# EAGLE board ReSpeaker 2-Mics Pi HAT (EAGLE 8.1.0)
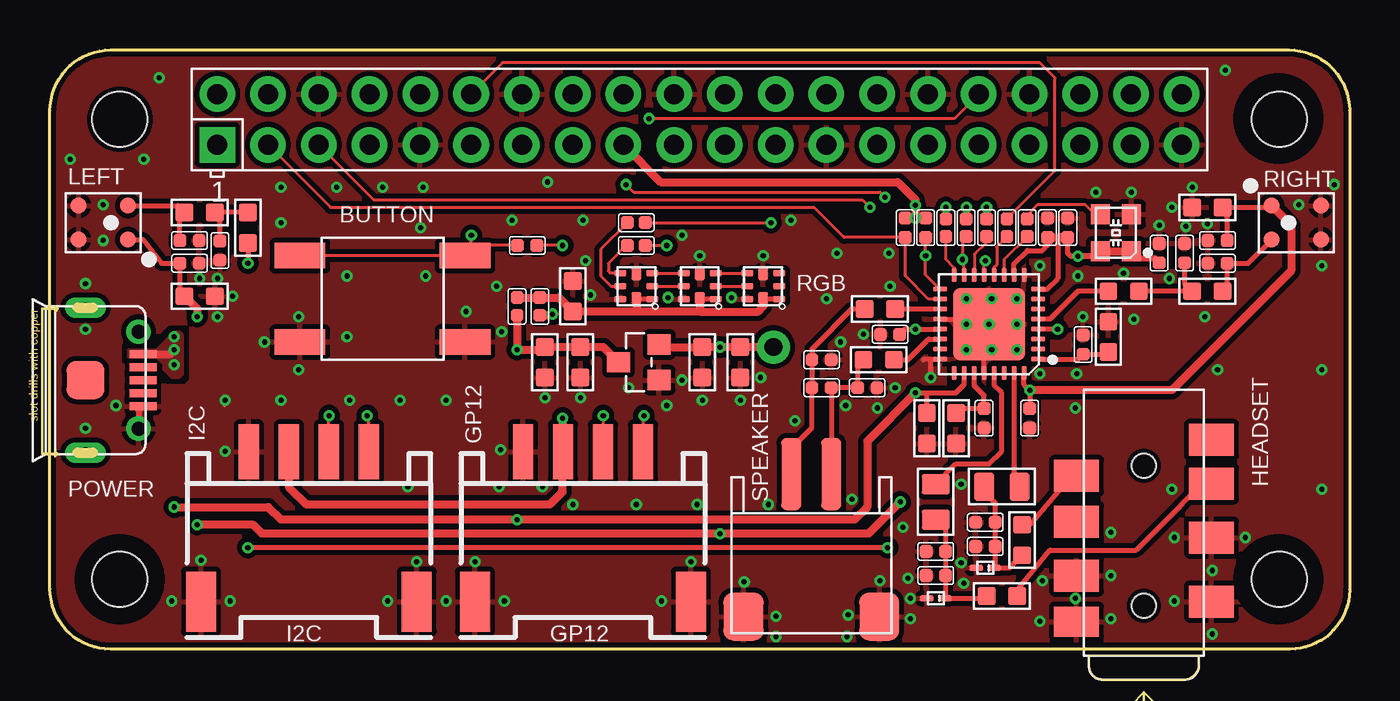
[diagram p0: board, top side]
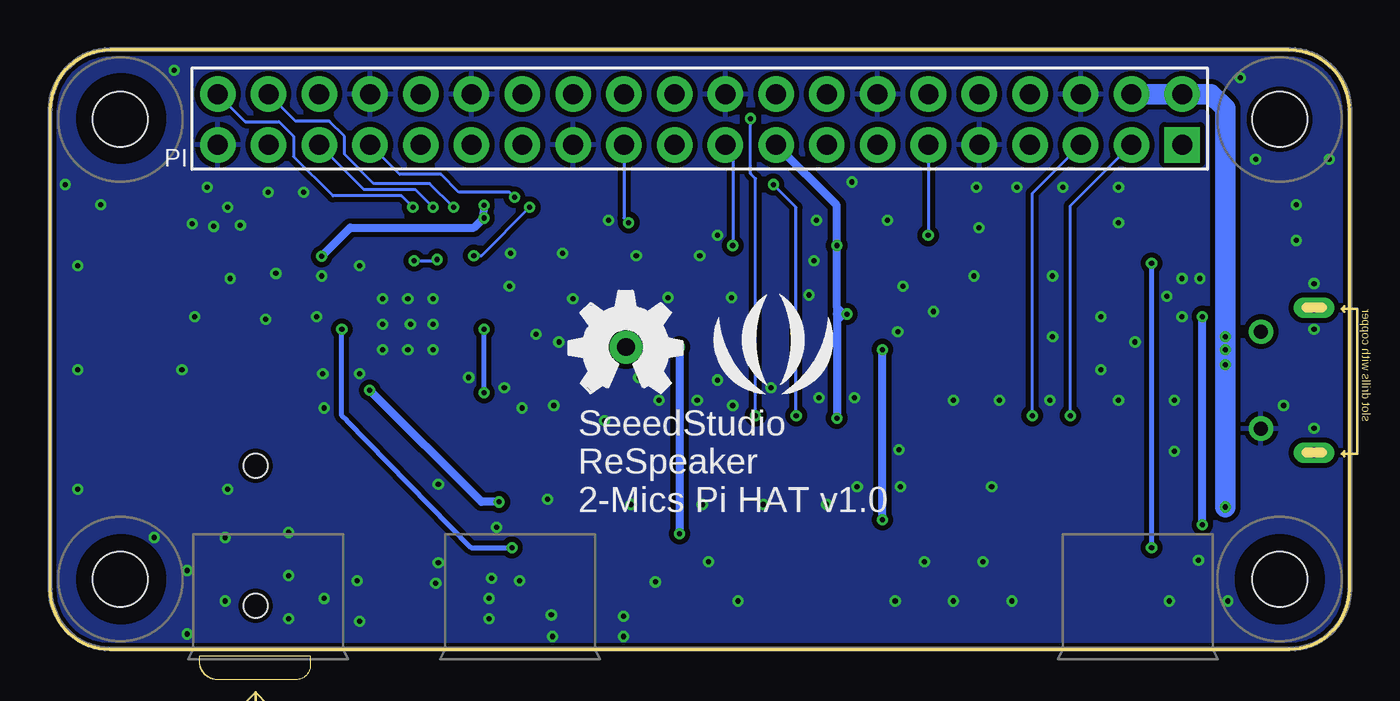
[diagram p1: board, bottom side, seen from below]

Size 65.02 x 29.97 mm. Coordinates in mm from the lower left corner, seen from the top.
Outline: 3.03,29.97 62,29.97 arc-90 65.02,26.95 65.02,2.98 arc-90 62.04,0 3.02,0 arc-90 0,3.02 0,26.94 arc-90 3.03,29.97
Copper layers (1*16): Top 0.035mm / dielectric 1.5mm / Bottom 0.035mm
Design rules "SeeedStudio_2layer_DRU_no_angle_20140221 *": minimum track width 6mil, minimum drill 10mil, track to track 6mil, track to pad 6mil, pad to pad 6mil, via to via 6mil, smd to smd 0mil, copper to edge 10mil, drill to drill 10mil, minimum pad ring 10mil, minimum via ring 6mil, stop-mask expansion 2mil, vias tented up to drill 25mil, thermal gap 10mil
tRestrict: area 59.5,24.5 to 63.5,28.5; area 59.5,1.5 to 63.5,5.5; area 1.5,1.5 to 5.5,5.5
bRestrict: area 59.5,24.5 to 63.5,28.5; area 59.5,1.5 to 63.5,5.5; area 1.5,1.5 to 5.5,5.5

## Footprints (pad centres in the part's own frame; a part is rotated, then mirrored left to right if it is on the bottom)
C0402 = smd 0.635 x 0.635: 1 0,0.484; 2 0,-0.484
C0603 = smd 0.889 x 0.889: 1 0,0.762; 2 0,-0.762
C0805 = smd 1.397 x 1.016: 1 0,0.889; 2 0,-0.889
RGB2020 = smd 0.6 x 0.3: 1 -0.8,0.65; 2 -0.8,0; 3 -0.8,-0.65; 4 0.8,-0.65; 5 0.8,0; 6 0.8,0.65 | smd 0.5 x 0.6: 7 0,-0.6; 8 0,0.6
SOD-923 = smd 0.7 x 0.3: 1 -0.45,0; 2 0.45,0
MICRO-USB5+5P-SMD-0.65-7.2X5.06MM = smd 0.4 x 1.35: 1 -1.3,2.875; 2 -0.65,2.875; 3 0,2.875; 4 0.65,2.875; 5 1.3,2.875 | smd 1.9 x 1.9: P1 0,0 | drill 0.508 pad 1.016 long: P3 -3.625,0; P4 3.625,0 | drill 0.7: P5 -2.425,2.65; P6 2.425,2.65
HW2-SMD-2.0-90D = smd 2 x 2.4: 3 3.4,-2.181; 4 -3.4,-2.181 | smd 1 x 3.6: + -1,4.953; - 1,4.953
HW4-SMD-2.0-90D = smd 1.01 x 2.74: 1 -3,-0.1; 2 -1,-0.1; 3 1,-0.1; 4 3,-0.1 | smd 1.5 x 3: SS1 -5.4,7.4; SS2 5.4,7.4
AUDIO8P-SMD-3.5-14.5X6.1X4.0MM = smd 1.6 x 2.25: 1 3.9,-3.375; 2 7.1,-3.375; 3 9.8,-3.375; 4 10.2,3.375; 6 5.2,3.375; 7 7.9,3.375; 8 12,-3.375 | smd 1.5 x 2.25: 5 2.9,3.375 | hole 1.2: 3.7,0; 10.7,0
SW4-SMD-6.0X6.0X5.0MM = smd 2.54 x 1.27: 1 -4.129,2.159; 2 -4.129,-2.159; 3 4.129,-2.159; 4 4.129,2.159
L0603 = smd 0.889 x 0.889: 1 -0.762,0; 2 0.762,0
MIC4-SMD-3.76X2.95MM = smd 0.8 x 0.8: 1 0.85,1.23; 2 0.85,-1.23; 3 -0.85,-1.23; 4 -0.85,1.23
RASPBERRYPI_BASTELSTUBE_V13_RASPI_BOARD_B+_FULL = drill 1 pad 1.778 square: 1 8.37,25.23 | drill 1 pad 1.778: 2 8.37,27.77; 3 10.91,25.23; 4 10.91,27.77; 5 13.45,25.23; 6 13.45,27.77; 7 15.99,25.23; 8 15.99,27.77; 9 18.53,25.23; 10 18.53,27.77; 11 21.07,25.23; 12 21.07,27.77; 13 23.61,25.23; 14 23.61,27.77; 15 26.15,25.23; 16 26.15,27.77; 17 28.69,25.23; 18 28.69,27.77; 19 31.23,25.23; 20 31.23,27.77; 21 33.77,25.23; 22 33.77,27.77; 23 36.31,25.23; 24 36.31,27.77; 25 38.85,25.23; 26 38.85,27.77; 27 41.39,25.23; 28 41.39,27.77; 29 43.93,25.23; 30 43.93,27.77; 31 46.47,25.23; 32 46.47,27.77; 33 49.01,25.23; 34 49.01,27.77; 35 51.55,25.23; 36 51.55,27.77; 37 54.09,25.23; 38 54.09,27.77; 39 56.63,25.23; 40 56.63,27.77 | hole 2.75: 3.5,3.5; 3.5,26.5; 61.5,3.5; 61.5,26.5
R0402 = smd 0.635 x 0.635: 1 0,0.484; 2 0,-0.484
R0402' = smd 0.635 x 0.635: 1 0,0.445; 2 0,-0.445
TP-D65/35MIL = drill 0.889 pad 1.651: P1 0,0
QFN32G-0.5-5X5MM = smd 0.7 x 0.25: 1 -2.45,1.75; 2 -2.45,1.25; 3 -2.45,0.75; 4 -2.45,0.25; 5 -2.45,-0.25; 6 -2.45,-0.75; 7 -2.45,-1.25; 8 -2.45,-1.75; 17 2.45,-1.75; 18 2.45,-1.25; 19 2.45,-0.75; 20 2.45,-0.25; 21 2.45,0.25; 22 2.45,0.75; 23 2.45,1.25; 24 2.45,1.75 | smd 0.25 x 0.7: 9 -1.75,-2.45; 10 -1.25,-2.45; 11 -0.75,-2.45; 12 -0.25,-2.45; 13 0.25,-2.45; 14 0.75,-2.45; 15 1.25,-2.45; 16 1.75,-2.45; 25 1.75,2.45; 26 1.25,2.45; 27 0.75,2.45; 28 0.25,2.45; 29 -0.25,2.45; 30 -0.75,2.45; 31 -1.25,2.45; 32 -1.75,2.45 | smd 3.6 x 3.6: 33 0,0
SOT-23 = smd 1.016 x 1.143: 1 -0.889,-1.016; 2 0.889,-1.016; 3 0,1.016
OSC4-SMD-2.5X2.0X0.8MM = smd 1 x 0.95: 1 -0.925,-0.775; 2 0.925,-0.775; 3 0.925,0.775; 4 -0.925,0.775

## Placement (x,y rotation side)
C1  100nF  [C0402]  42.04,15.75 90 top
C2  10uF  [C0603]  26.16,17.65 180 top
C3  10uF  [C0603]  43.88,11.05 0 top
C4  100nF  [C0402]  46.74,11.56 180 top
C5  10uF  [C0603]  45.34,11.05 0 top
C6  100nF  [C0402]  50.93,21.08 0 top
C7  100nF  [C0402]  51.69,15.24 180 top
C8  10uF  [C0603]  52.96,15.62 0 top
C9  100pF  [C0402]  40.89,13.08 270 top
C10  10uF  [C0603]  7.49,17.65 270 top
C11  100nF  [C0402]  58.42,20.45 90 top
C12  10uF  [C0603]  53.72,17.91 270 top
C13  10uF  [C0603]  24.77,14.35 180 top
C14  10uF  [C0603]  26.54,14.35 180 top
C15  10uF  [C0603]  34.54,14.35 180 top
C16  10uF  [C0603]  32.64,14.35 180 top
C17  100nF  [C0402]  49.02,11.56 180 top
C18  100nF  [C0402]  49.91,21.08 0 top
C19  33pF  [C0402]  58.42,19.3 90 top
C20  33pF  [C0402]  56.77,19.81 0 top
C21  10uF  [C0603]  57.91,22.1 90 top
C23  100nF  [C0402]  55.5,19.81 0 top
C31  680nF DNP  [C0402]  38.61,13.08 270 top
C32  100pF  [C0402]  38.61,14.48 270 top
C36  10uF  [C0603]  9.91,21.08 0 top
C37  100nF  [C0402]  6.98,19.3 270 top
C38  33pF  [C0402]  6.98,20.45 270 top
C39  33pF  [C0402]  8.51,19.94 180 top
C90  100uF 10V  [C0805]  44.32,7.37 0 top
C91  100uF 10V  [C0805]  47.62,8.13 270 top
C92  100pF  [C0402]  46.8,6.35 90 top
C93  100pF  [C0402]  44.32,4.89 90 top
D1  APA102-2020  [RGB2020]  29.34,18.16 180 top
D2  APA102-2020  [RGB2020]  32.51,18.16 180 top
D3  APA102-2020  [RGB2020]  35.69,18.16 180 top
D8  DF2S6.8FS  [SOD-923]  46.8,4.06 180 top
D9  DF2S6.8FS  [SOD-923]  44.32,2.54 180 top
FR1  SEEEDSTUDIO-OPEN-SCH-FRAME  [SEEEDSTUDIO-PCB-FRAME]  not placed on the board
FR8  SEEEDSTUDIO-OPEN-SCH-FRAME  [SEEEDSTUDIO-PCB-FRAME]  not placed on the board
J1  [MICRO-USB5+5P-SMD-0.65-7.2X5.06MM]  1.78,13.46 270 top
J2  JST-2P  [HW2-SMD-2.0-90D]  38.1,3.81 0 top
J3  [HW4-SMD-2.0-90D]  12.95,9.78 180 top
J4  [HW4-SMD-2.0-90D]  26.67,9.78 180 top
J9  DNP AUDIO-JACK-8P-SMD  [AUDIO8P-SMD-3.5-14.5X6.1X4.0MM]  54.74,-1.52 90 top
K1  [SW4-SMD-6.0X6.0X5.0MM]  16.64,17.53 0 top
L1  MPZ1608D101BTA00  [L0603]  47.62,2.67 0 top
L2  BLM18BD252SN1  [L0603]  57.91,17.91 180 top
L4  MPZ1608D101BTA00  [L0603]  48.64,5.46 90 top
L6  120R  [L0603]  41.47,14.48 180 top
L7  120R  [L0603]  41.53,17.02 180 top
L8  BLM18BD252SN1  [L0603]  7.49,21.84 0 top
MIC1  SAO-3729-M-42-008  [MIC4-SMD-3.76X2.95MM]  2.67,21.34 270 top
MIC2  SAO-3729-M-42-008  [MIC4-SMD-3.76X2.95MM]  62.36,21.34 90 top
PI  RPI-ZERO  [RASPBERRYPI_BASTELSTUBE_V13_RASPI_BOARD_B+_FULL]  0,0 0 top
R1  10k  [R0402]  46.8,5.14 90 top
R2  10R  [R0402']  29.34,20.19 90 top
R3  10R  [R0402']  29.34,21.34 90 top
R4  10k  [R0402]  23.88,20.19 90 top
R6  10k  [R0402]  43.81,21.08 180 top
R7  0R  [R0402']  23.37,17.15 0 top
R8  10k  [R0402]  42.8,21.08 180 top
R9  DNP  [R0402']  24.51,17.15 0 top
R10  10R  [R0402']  48.89,21.08 180 top
R11  10R  [R0402']  47.88,21.08 180 top
R12  10R  [R0402']  46.86,21.08 180 top
R13  10R  [R0402']  45.85,21.08 180 top
R19  10R  [R0402']  44.83,21.08 180 top
R39  10k  [R0402]  44.32,3.68 90 top
TP1  [TP-D65/35MIL]  36.19,15.11 0 top
U2  WM8960  [QFN32G-0.5-5X5MM]  46.99,16.26 180 top
U4  XC6206 3.3V  [SOT-23]  29.46,14.35 90 top
U$13  [SEEED-SILK-280*268MIL]  28.83,14.48 0 bottom
U$22  [OSHW_FILLX200_NOTEXT_TNAME]  39.05,12.83 0 bottom
X2  24MHz 306020014  [OSC4-SMD-2.5X2.0X0.8MM]  53.34,20.83 90 top

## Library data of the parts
C1-C21 C23 C31 C32 C36-C39 C90-C93 D1-D3 D8 D9 K1 L1 L2 L4 L6-L8 R1 R4 R6 R8 R39 TP1 X2 = Discrete-new
FR1 FR8 = moudle-new
J1-J4 J9 MIC1 MIC2 = Connector-new
PI = RPI-Zero
R2 R3 R7 R9-R13 R19 = C-R-package test
U2 U4 = IC-new
U$13 U$22 = Logo

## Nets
$123: C90.1 U2.29
$124: C91.1 U2.31
AIN1P: U2.3
AIN2P: U2.6
AVDD_3V3: C10.2 C11.2 C15.2 C16.2 C17.2 C21.2 C37.2 MIC1.1 MIC2.1 TP1.P1 U2.32 U4.2
GND: C1.1 C2.2 C3.2 C4.1 C5.2 C6.1 C7.2 C8.1 C9.1 C10.1 C11.1 C13.1 C14.1 C15.1 C16.1 C17.1 C18.1 C19.1 C20.1 C21.1 C23.1 C32.1 C37.1 C38.1 C39.1 C92.1 C93.1 D1.6 D1.7 D2.6 D2.7 D3.6 D3.7 D8.2 D9.2 J1.5 J1.P6 J2.3 J2.4 J3.4 J3.SS1 J3.SS2 J4.4 J4.SS1 J4.SS2 J9.1 J9.2 J9.5 J9.6 K1.2 K1.3 MIC1.2 MIC1.3 MIC2.2 MIC2.3 PI.6 PI.9 PI.14 PI.20 PI.25 PI.30 PI.34 PI.39 R1.1 R39.1 U2.9 U2.20 U2.24 U2.28 U2.33 U4.1 X2.2
GPIO12: J4.1 PI.32
GPIO13: J4.2 PI.33
GPIO17: K1.1 K1.4 PI.11 R4.1
HP_L: C91.2 C92.2 D8.1 L4.1 R1.2
HP_R: C90.2 C93.2 D9.1 L1.1 R39.2
I2C_SCL: J3.1 PI.5 R6.1 U2.17
I2C_SDA: J3.2 PI.3 R8.1 U2.18
I2S_ADC: PI.38 R19.2
I2S_CLK: PI.12 R11.2
I2S_DAC: PI.40 R12.2
I2S_LRCLK: PI.35 R13.2
LINPUT1: C36.2 U2.4
MCLK: R10.2 X2.3
MICBIAS: C7.1 C8.2 U2.1
N$1: D1.2 D2.5
N$2: D1.4 R2.1
N$3: C12.1 C20.2 L2.2
N$4: D1.3 D2.4
N$5: D1.5 R3.1
N$6: C38.2 L8.1 MIC1.4
N$7: C19.2 L2.1 MIC2.4
N$8: D2.2 D3.5
N$9: L6.1 U2.22
N$10: R12.1 U2.14
N$11: D2.3 D3.4
N$12: L7.1 U2.19
N$14: J9.3 L1.2
N$15: D3.2
N$19: D3.3
N$24: C36.1 C39.2 L8.2
N$34: R19.1 U2.16
N$35: R13.1 U2.13 U2.15
N$36: R11.1 U2.12
N$37: R10.1 U2.11
N$40: C9.2 C31.1 J2.- L6.2
N$47: C31.2 C32.2 J2.+ L7.2
N$57: J9.4 L4.2
RINPUT1: C12.2 U2.5
SPI_MOSI: PI.19 R2.2
SPI_SCLK: PI.23 R3.2
UART_RXD0: PI.10
UART_TXD0: PI.8
VDD_3V3: C6.2 C18.2 C23.2 J3.3 J4.3 PI.17 R4.2 R6.2 R8.2 R9.2 U2.8 U2.10 X2.1 X2.4
VDD_5V: C1.2 C3.1 C13.2 C14.2 J1.1 PI.2 PI.4 R7.2 U2.21 U2.26 U4.3
VDD_LED: C2.1 D1.1 D1.8 D2.1 D2.8 D3.1 D3.8 R7.1 R9.1
VMID: C4.2 C5.1 U2.27

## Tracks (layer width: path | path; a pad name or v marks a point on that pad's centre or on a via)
$123
  Top 0.254: U2.29 47.24,13.21 47.62,12.83 47.62,9.91 46.99,9.27 45.34,9.27 C90.1
$124
  Top 0.254: U2.31 48.24,8.4 C91.1
AVDD_3V3  (via drill 0.25 pad 0.51)
  Top 0.152: 33.65,15.11 v33.53,15.11
  Top 0.254: C17.2 v49.02,12.95 48.74,13.24 U2.32 | C11.2 58.9,21.61 C21.2 61.04,22.1 MIC2.1 | MIC1.1 4.66,20.49 5.59,19.3 C37.2 6.5,17.88 C10.2
  Top 0.406: v33.53,15.11 C16.2 30.61,15.11 U4.2 | 33.65,15.11 C15.2 TP1.P1 | v42.54,7.37 40.96,5.78 v33.53,5.78 10.61,5.78 10.17,6.22 v7.37,6.22 | MIC2.1 62.1,21.21 62.1,18.92 56.13,12.95 v49.02,12.95 | C10.2 7.37,17.02 v7.37,16.64
  Bottom 0.406: v33.53,15.11 v33.53,5.78 | v42.54,7.37 43.43,7.37 v49.02,12.95 | v7.37,6.22 v7.37,16.64
GND  (via drill 0.25 pad 0.51)
  Top 0.152: 8.73,12.16 8.76,12.19
  Top 0.254: 43.69,14.48 43.72,14.51 44.07,14.51 | U2.28 46.74,14.61 v47.12,14.99 | U2.20 45.6,16.51 v45.85,16.26 | 44.07,14.51 U2.24 | v44.07,13.59 44.07,14.51
  Top 0.305: J1.5 4.43,11.94 J1.P6
  other vias: 8.76,12.45 3.3,12.19 8.76,9.91 22.54,9.97 19.81,12.45 24.77,12.57 26.54,12.57 28.96,13.08 31.62,13.46 32.51,19.69 35.69,19.69 35.56,13.59 34.54,12.45 32.64,12.45 41.4,12.06 42.29,13.08 45.85,17.53 47.12,17.53 48.39,17.53 48.39,14.99 45.85,14.99 48.39,16.26 46.99,16.26 49.53,19.18 51.69,16.64 54.23,16.51 63.63,19.18 64.26,23.24 62.48,22.23 57.15,23.11 56.13,22.1 54.1,22.86 57.78,16.64 55.5,21.21 56.26,5.59 56.26,2.41 58.17,0.76 58.17,3.94 59.82,5.59 53.09,3.68 51.31,2.54 53.09,1.52 49.53,1.4 49.66,3.43 45.72,3.3 45.59,4.32 45.59,8.25 42.67,6.1 42.93,3.56 43.05,2.54 43.05,1.52 30.61,2.41 22.73,2.41 19.81,2.41 16.89,2.41 9.02,2.41 6.1,2.41 1.78,11.05 1.78,16 1.78,18.29 2.67,20.45 2.67,22.23 1.02,24.51 9.14,17.65 8.38,16.64 7.49,18.54 8.38,18.54 11.56,12.45 26.16,7.24 32.38,7.24 35.94,7.24 30.86,12.19 30.92,17.59 34.1,17.59 27.05,17.72 26.8,19.43 26.67,21.46 31.62,20.7 37.08,21.46 40.13,7.49 39.81,12.19 40.7,15.75 39.56,15.37 57.91,21.27 56.83,21.15 5.46,28.58 18.67,23.11 24.89,23.37 18.54,21.08 22.35,18.16 22.61,15.88 14.86,15.62 12.45,16.64 12.45,13.97 14.99,12.45 63.63,8 63.63,13.97 58.8,28.96 52.32,22.86 58.42,13.97 49.53,13.78 53.09,5.84 56.13,8 39.88,0.64 36.32,0.64 17.91,8.13 22.48,8.13 17.53,12.45 4.7,24.51 18.8,18.67 20.83,16.89 10.73,15.37 56.01,18.54 51.43,18.67 53.72,18.8 37.27,11.43 41.97,19.81 42.04,18.16 39.37,19.81 38.86,17.53 29.34,7.24 24.64,8.13 16.64,23.11 14.35,23.11 11.56,23.11 11.56,21.34 14.86,18.67 23.11,21.46 51.37,13.78 51.31,12.06 18.35,4.38 21.27,4.38 32.07,4.38 7.56,4.45 34.73,3.37 39.94,1.71 36.32,1.65 41.53,3.43
  pour Top: -25.27,23.24 -25.27,21.34 -22.73,21.34 -22.73,23.24
  pour Top (isolate 0.254, rank 4): 0,0 65.53,0 66.8,0 66.8,30.23 0,30.23
  pour Bottom (isolate 0.254, rank 4): -0.13,0 65.41,0 66.67,0 66.67,30.23 -0.13,30.23
GPIO12  (via drill 0.25 pad 0.51)
  Top 0.152: PI.32 45.24,26.54 v29.97,26.54 | v29.72,11.68 29.67,11.64 J4.1
  Bottom 0.152: v29.72,11.68 29.72,23.53 29.97,23.79 v29.97,26.54
GPIO13  (via drill 0.25 pad 0.51)
  Top 0.152: v27.69,11.68 27.67,11.67 J4.2 | v41.78,22.61 41.53,22.86 29.21,22.86 v28.83,23.24
  Bottom 0.152: PI.33 47.53,23.75 45.47,23.75 44.58,22.86 42.04,22.86 v41.78,22.61 | v27.69,11.68 27.69,22.1 v28.83,23.24
GPIO17  (via drill 0.25 pad 0.51)
  Top 0.152: K1.4 K1.1 | 21.08,20 arc-90 K1.4 | 21.08,20 v21.08,20.7 | 20.87,19.58 K1.4 | R4.1 21.27,20.19 21.08,20
  Bottom 0.152: PI.11 21.07,20.7 v21.08,20.7
HP_L
  Top 0.254: C91.2 46.74,7.87 46.86,7.75 46.99,7.62 47.28,7.33 C92.2 R1.2 47.28,4.1 D8.1 48.01,4.06 L4.1
HP_R
  Top 0.254: C90.2 44.81,5.99 C93.2 R39.2 44.81,2.57 D9.1 46.74,2.54 L1.1
I2C_SCL  (via drill 0.25 pad 0.51)
  Top 0.152: J3.1 15.95,11.35 15.94,11.37 15.94,11.62 v15.88,11.68 | U2.17 43.81,18.73 v43.81,19.69 R6.1 | PI.5 16.2,22.48 40.64,22.48 v41.02,22.1
  Bottom 0.152: v15.88,11.68 15.88,22.8 PI.5 | v43.81,19.69 43.43,19.69 v41.02,22.1
I2C_SDA  (via drill 0.25 pad 0.51)
  Top 0.152: U2.18 43.96,17.51 42.8,18.67 R8.1 39.73,20.6 38.23,22.1 14.04,22.1 PI.3 | J3.2 13.95,11.67
  Top 0.254: v13.97,11.68 13.95,11.67
  Bottom 0.152: v13.97,11.68 13.97,22.17 PI.3
I2S_ADC  (via drill 0.25 pad 0.51)
  Top 0.152: R19.2 v44.83,22.1
  Bottom 0.152: PI.38 52.74,26.42 51.05,26.42 50.29,25.65 50.29,24.77 48.82,23.29 46.02,23.29 v44.83,22.1
I2S_CLK
  Top 0.152: PI.12 22.64,29.34 49.53,29.34 50.29,28.58 50.29,23.94 R11.2
I2S_DAC  (via drill 0.25 pad 0.51)
  Top 0.152: R12.2 v46.86,22.1
  Bottom 0.152: PI.40 55.24,26.38 53.56,26.38 52.83,25.65 52.83,24.64 50.86,22.67 47.43,22.67 v46.86,22.1
I2S_LRCLK  (via drill 0.25 pad 0.51)
  Top 0.152: R13.2 v45.85,22.1
  Bottom 0.152: PI.35 49.31,22.99 46.74,22.99 v45.85,22.1
LINPUT1  (via drill 0.25 pad 0.51)
  Top 0.254: C36.2 v9.91,19.3 | v50.42,16 U2.4 | v41.91,5.08 v9.91,5.08
  Bottom 0.254: v9.91,19.3 v9.91,5.08 | v41.91,5.08 43.94,5.08 50.16,11.43 50.42,11.68 v50.42,16
MCLK
  Top 0.152: R10.2 48.89,21.72 49.4,22.23 51.82,22.23 52.54,21.5 X2.3
MICBIAS
  Top 0.254: C8.2 52.73,14.76 C7.1 51.44,14.51 U2.1
N$1
  Top 0.152: D1.2 D2.5
N$2
  Top 0.152: D1.4 28.05,18.81 27.94,18.92 27.94,19.3 28.83,20.19 R2.1
N$3
  Top 0.254: C20.2 56.77,18.29 L2.2 C12.1
N$4
  Top 0.152: D1.3 D2.4
N$5
  Top 0.152: D1.5 28.07,18.16 27.56,18.67 27.56,20 R3.1
N$6
  Top 0.254: MIC1.4 6.39,22.19 L8.1 6.5,21.61 C38.2
N$7
  Top 0.254: L2.1 58.9,18.14 C19.2 59.94,19.3 MIC2.4
N$8
  Top 0.152: D2.2 D3.5
N$9
  Top 0.254: U2.22 43.95,15.51 42.93,14.48 L6.1
N$10
  Top 0.152: R12.1 46.86,20.34 46.29,19.77 46.29,18.76 U2.14
N$11
  Top 0.152: D2.3 D3.4
N$12
  Top 0.254: U2.19 42.3,17.01 L7.1
N$14
  Top 0.254: L1.2 48.39,2.92 50.04,4.95 54.36,4.95 56.51,7.11 56.64,7.24 57.68,8.28 J9.3
N$24
  Top 0.254: C39.2 8.51,21.59 L8.2 C36.1
N$34
  Top 0.152: U2.16 45.24,19.09 44.83,19.49 R19.1
N$35  (via drill 0.25 pad 0.51)
  Top 0.152: U2.13 46.74,19.37 v46.8,19.43 | U2.15 45.74,19.41 v45.66,19.49 45.66,20.45 R13.1
  Bottom 0.152: v46.8,19.43 45.72,19.43 v45.66,19.49
N$36
  Top 0.152: U2.12 47.24,19.11 47.37,19.24 47.37,20.13 R11.1
N$37
  Top 0.152: R10.1 47.74,19.48 U2.11
N$40
  Top 0.254: L6.2 40.41,14.18 C9.2 C31.1 J2.-
N$47
  Top 0.254: L7.2 40.13,17.02 38.12,15.01 C32.2 C31.2 38.12,11.07 37.1,10.05 J2.+
N$57
  Top 0.254: L4.2 49.02,6.22 51.09,8.68 J9.4
RINPUT1
  Top 0.254: U2.5 50.03,16.51 51.43,17.91 C12.2
SPI_MOSI  (via drill 0.25 pad 0.51)
  Top 0.152: R2.2 v30.86,20.19
  Bottom 0.152: PI.19 30.86,24.86 v30.86,20.19
SPI_SCLK  (via drill 0.25 pad 0.51)
  Top 0.152: R3.2 v36.07,21.34
  Bottom 0.152: v36.07,21.34 36.31,21.58 PI.23
VDD_3V3  (via drill 0.25 pad 0.51)
  Top 0.152: v25.65,20.19 R4.2
  Top 0.254: U2.8 49.88,18.01 50.42,18.54 50.42,20.6 | U2.10 48.24,19.28 48.89,19.94 49.66,19.94 49.91,20.19 C18.2 | v51.43,19.65 51.09,19.65 50.93,19.81 C6.2
  Top 0.305: X2.4 52.31,19.65 v51.43,19.65 | C23.2 55.27,19.56 54.46,19.56 X2.1
  Top 0.406: X2.4 X2.1 | C18.2 50.42,20.6 C6.2 | J3.3 11.95,8.11 12.83,7.24 25.02,7.24 25.65,7.87 25.65,9.86 J4.3 25.67,11.54 v25.65,11.56 | v43.31,21.57 R8.2 | v43.31,21.57 R6.2 | v43.31,21.57 v43.31,22.2 43.31,22.48 42.42,23.37 30.55,23.37 PI.17 | R9.2 25.15,16.7 v25.15,16.76
  Bottom 0.152: 25.65,17.15 25.53,17.15 v25.15,16.76 25.53,16.38
  Bottom 0.406: v51.43,19.65 50,21.08 43.81,21.08 43.33,21.57 v43.31,22.2 | 25.65,16.76 v25.65,11.56 | 25.65,16.76 25.65,17.15 v25.65,20.19 25.65,22.19 PI.17 | 25.65,16.76 v25.15,16.76
VDD_5V  (via drill 0.25 pad 0.51)
  Top 0.254: U2.26 45.74,13.23 45.34,12.83 43.94,12.83 | C1.2 42.78,16.01 v43.31,16.01 U2.21 | v43.31,12.83 43.94,12.83 | C3.1 43.88,12.76 43.94,12.83
  Top 0.406: C13.2 C14.2 27.69,15.11 U4.3 | J1.1 6,14.76 v6.22,14.99 | C13.2 24.64,14.99 v23.37,14.99 R7.2 | 24.64,15.24 C13.2 | v6.22,7.11 10.92,7.11 11.56,6.48 v23.37,6.48 40.26,6.48 40.89,7.11 40.89,10.41 v43.31,12.83
  Bottom 0.254: v43.31,12.83 v43.31,16.01
  Bottom 0.406: v23.37,6.48 v23.37,14.99
  Bottom 1.016: PI.4 PI.2 6.94,27.77 6.22,27.05 v6.22,14.99 v6.22,7.11
  other vias: 6.22,15.62 6.22,14.22
  pour Top (no thermals): 3.94,14.99 5.33,14.99 6.22,15.88 6.48,15.88 6.6,15.75 6.6,13.72 6.48,13.59 6.1,13.59 5.71,13.97 5.71,14.22 5.33,14.61 3.94,14.61
VDD_LED
  Top 0.254: D1.1 29.39,17.51 | D2.1 32.56,17.51 | D3.1 35.74,17.51
  Top 0.406: 35.74,17.51 D3.8 35.69,17.15 35.43,16.89 32.51,16.89 | 32.56,17.51 D2.8 32.51,16.89 | R7.1 R9.1 25.46,17.59 C2.1 29.34,16.89 | 29.39,17.51 D1.8 29.34,16.89 | 32.51,16.89 29.34,16.89
VMID
  Top 0.254: U2.27 46.24,13.2 46.74,12.7 C4.2 45.57,12.04 C5.1

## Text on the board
tPlace: LEFT | RIGHT | BUTTON | RGB | I2C | GP12 | POWER | HEADSET | SPEAKER | I2C | GP12
bPlace: PI | SeeedStudio / ReSpeaker / 2-Mics Pi HAT v1.0

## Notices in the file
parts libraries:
moudle-new: This work is licensed under the Creative Commons Attribution 4.0 International License.
To view a copy of this license,visit:
http://creativecommons.org/licenses/by-sa/4.0
